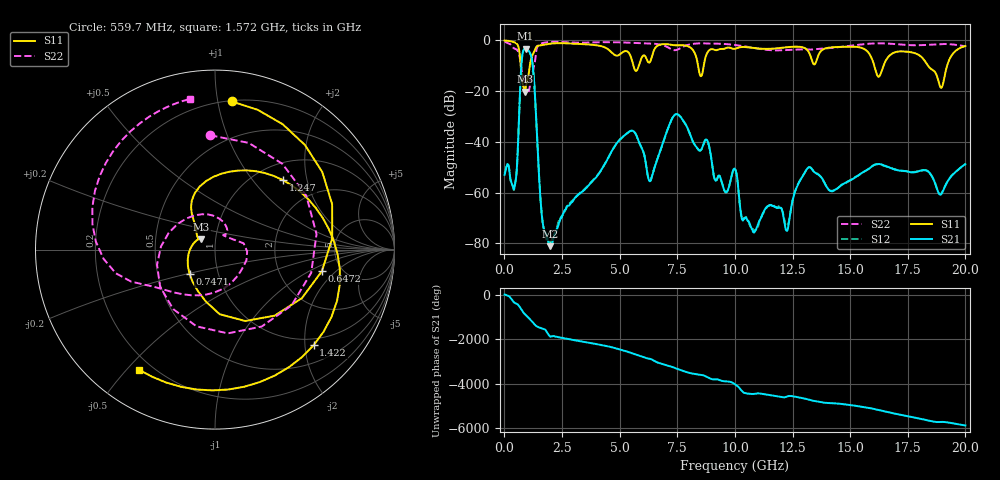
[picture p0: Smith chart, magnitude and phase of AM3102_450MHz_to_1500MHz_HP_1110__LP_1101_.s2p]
!Agilent Technologies,E8364B,MY43040894,A.07.50.67
!Agilent E8364B: A.07.50.67
!Date: Thursday, January 11, 2018 06:45:44
!Correction: S11(Full 2 Port(1,2))
!S21(Full 2 Port(1,2))
!S12(Full 2 Port(1,2))
!S22(Full 2 Port(1,2))
!S2P File: Measurements: S11, S21, S12, S22:
# Hz S  dB  R 50
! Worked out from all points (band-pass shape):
!   1601 points, 10 MHz to 20 GHz, reference 50 ohm
!   highest |S21| = -3.33 dB at 922 MHz (marker M1); lowest = -81.1 dB at 1.984 GHz (marker M2)
!   |S21| within 3 dB of the highest: 772.4 MHz to 1.166 GHz (393.5 MHz wide, 40.6 % of centre)
!   lowest |S11| = -20.3 dB at 884.6 MHz (marker M3), VSWR 1.21, Z = 42.7 + j5.16 ohm
!   |S11| at or under -10 dB: 705 MHz to 1.103 GHz (397.5 MHz wide, 44 % of centre); 16.05 GHz to 16.45 GHz (402.7 MHz wide, 2.48 % of centre); 18.38 GHz to 19.21 GHz (832.5 MHz wide, 4.43 % of centre)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
!   |S22| runs from -20.7 to -0.5 dB; largest |S21 - S12| = 0.00053
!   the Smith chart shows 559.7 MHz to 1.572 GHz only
!   S11 on the Smith chart (normalised r, x): 559.7 MHz: 0.21, +1.10; 647.2 MHz: 3.55, -1.35; 747.1 MHz: 0.73, -0.20; 1.247 GHz: 1.32, +1.45; 1.422 GHz: 0.85, -2.19; 1.572 GHz: 0.15, -0.54
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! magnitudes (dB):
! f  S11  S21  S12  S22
! 10 MHz  -0.1  -53.0  -52.4  -0.5
! 559.7 MHz  -1.6  -47.5  -47.7  -3.9
! 647.2 MHz  -4.3  -27.2  -27.2  -6.0
! 747.1 MHz  -14.2  -8.6  -8.6  -11.9
! 884.6 MHz  -20.3  -3.4  -3.4  -17.2
! 922 MHz  -18.7  -3.3  -3.3  -20.3
! 1.247 GHz  -5.3  -11.4  -11.4  -11.9
! 1.422 GHz  -2.3  -38.7  -38.7  -2.8
! 1.572 GHz  -2.0  -63.2  -63.5  -1.4
! 1.984 GHz  -1.4  -81.1  -79.9  -0.7
! 3.346 GHz  -1.5  -59.7  -59.6  -1.0
! 5.445 GHz  -5.6  -35.8  -35.9  -1.0
! 6.294 GHz  -8.8  -55.5  -55.4  -1.3
! 6.682 GHz  -2.0  -45.6  -45.7  -1.6
! 7.494 GHz  -2.0  -29.1  -29.1  -3.8
! 10.01 GHz  -3.4  -50.7  -50.7  -1.9
! 10.83 GHz  -3.1  -75.7  -75.0  -3.1
! 12.27 GHz  -2.7  -74.9  -72.7  -3.9
! 13.34 GHz  -8.0  -50.7  -50.7  -3.7
! 16.68 GHz  -6.4  -50.0  -50.0  -1.3
! 18.95 GHz  -18.7  -60.6  -60.4  -1.5
! 20 GHz  -2.3  -48.9  -48.8  -2.3
